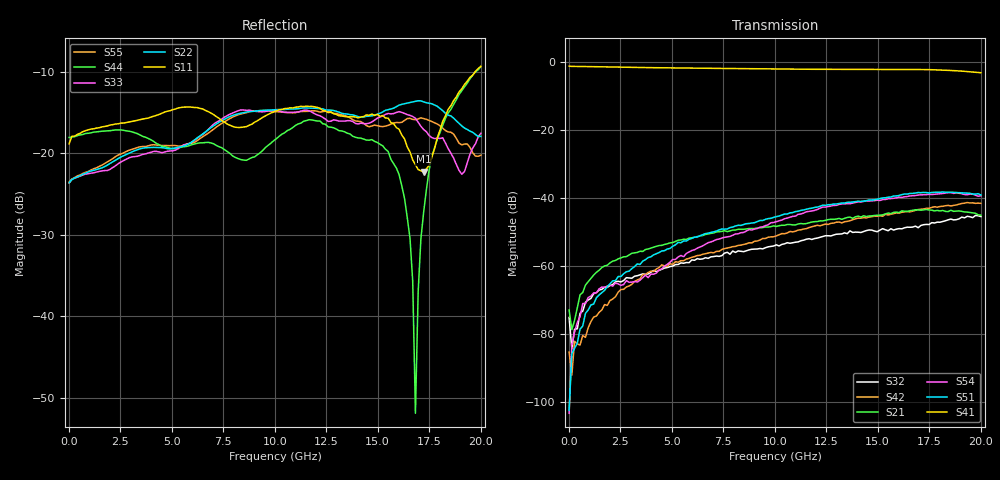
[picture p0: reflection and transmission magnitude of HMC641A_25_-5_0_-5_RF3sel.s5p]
! Device:  HMC641A
! Description: GaAs MMIC SP4T NON-REFLECTIVE
! Frequency:  0.01 -  18 GHz
! Ports:
! RFC = Port 1
! RF1 = Port 2
! RF2 = Port 3
! RF3 = Port 4
! RF4 = Port 5
! State: RF3 selected
! Vss:  -5 Volts
! Control A  0 Volts
! Control B:  -5 Volts
! Temperature = +25 C
! Data: Data was collected using a calibrated network analyzer.
!  The reference plane is the edge of the device.
! Note: Analog Devices supplies this data as a sample of measured data for this product.
!  Your particular data for this product may vary.
!  Analog Devices reserves the right to change this data at anytime
# Hz S DB R 50.0
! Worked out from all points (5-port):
!   152 points, 10 MHz to 20.01 GHz, reference 50 ohm
!   strongest paths, dB at 10 MHz, 5.043 GHz, 10.08 GHz, 15.11 GHz, 20.01 GHz:
!     S41: -1.1, -1.6, -1.9, -2.1, -3.1
!     S51: -102.6, -54.2, -45.5, -40.1, -39.1
!     S54: -103.4, -58.1, -46.9, -40.7, -39.3
!     S21: -73.0, -53.1, -48.4, -45.0, -45.0
!     S42: -85.4, -59.5, -51.1, -45.2, -41.6
!     S32: -75.2, -60.0, -53.8, -49.4, -45.4
!   lowest |S11| = -22.3 dB at 17.23 GHz (marker M1), VSWR 1.17, Z = 42.9 - j0.453 ohm
!   |S11| at or under -10 dB: start of sweep to 19.74 GHz
